| IBIS file stm32h562_563_573_lqfp64.ibs
[IBIS ver] 4.2
[File name] stm32h562_563_573_lqfp64.ibs
[File Rev] 1.1
[Date] 07-05-2024
[Source] Data Created at STMicroelectronics
[Notes]  File originated from ELDO simulations.
[Disclaimer]  This information is for modeling purpose only and is
   not guaranteed. The information is subject to change without
   notice.
[Copyright] Copyright 2024 STMicroelectronics Inc.
|   Component stm32h562_563_573_lqfp64
[Component] stm32h562_563_573_lqfp64
[Manufacturer] STMicroelectronics
[Package]
| variable   typ   min   max
R_pkg  0  NA  NA
L_pkg  0  NA  NA
C_pkg  0  NA  NA
[Pin]   signal_name   model_name
1  VBAT  power
2  PC13  io8_ft_i3c_spi
3  PC14-OSC32_IN  io8_ft_i3c_spi
4  PC15-OSC32_OUT  io8_ft_i3c_spi
5  PH0-OSC_IN  io8_ft_i3c_spi
6  PH1-OSC_OUT  io8_ft_i3c_spi
7  NRST  ioreset_ft_v33
8  PC0  io8_ft_spi
9  PC1  io8_ft_spi
10  PC2  io8_ft_spi
11  PC3  io8_ft_spi
12  VSSA  nc
13  VDDA  nc
14  PA0  io8_ft_spi
15  PA1  io8_ft_spi_tamp
16  PA2  io8_ft_spi
17  PA3  io8_ft_spi
18  VSS  gnd
19  VDD  power
20  PA4  io8_ft_spi
21  PA5  io8_ft_spi
22  PA6  io8_ft_spi
23  PA7  io8_ft_spi
24  PC4  io8_ft_spi
25  PC5  io8_ft_spi
26  PB0  io8_ft_spi
27  PB1  io8_ft_spi
28  PB2  io8_ft_i3c_spi
29  PB10  io8_ft_i3c_spi
30  VCAP  nc
31  VSS  gnd
32  VDD  power
33  PB12  io8_ft_i3c_spi
|34  PB13  io8usb_ft_pd
|35  PB14  io8usb_ft_pd
34 PB13 nc
35 PB14 nc
36  PB15  io8_ft_spi
37  PC6  io8_ft_i3c_spi
38  PC7  io8_ft_i3c_spi
39  PC8  io8_ft_i3c_spi
40  PC9  io8_ft_i3c_spi
41  PA8  io8_ft_i3c_spi
42  PA9  io8_ft_i3c_spi
43  PA10  io8_ft_i3c_spi
44  PA11  io8usb_ft_i3c_spi_phy
45  PA12  io8usb_ft_i3c_spi_phy
46  PA13  io8_ft_i3c_spi
47  VSS  gnd
48  VDD  power
49  PA14  io8_ft_i3c_spi
50  PA15  io8_ft_i3c_spi
51  PC10  io8_ft_i3c_spi
52  PC11  io8_ft_i3c_spi
53  PC12  io8_ft_i3c_spi
54  PD2  io8_ft_i3c_spi
55  PB3  io8_ft_i3c_spi
56  PB4  io8_ft_i3c_spi
57  PB5  io8_ft_i3c_spi
58  PB6  io8_ft_i3c_spi
59  PB7  io8_ft_i3c_spi
60  BOOT0  vpphv
61  PB8  io8_ft_i3c_spi
62  VCAP  nc
63  VSS  gnd
64  VDD  power
[Package Model]   484-lqfp-10x10-64-ldo-221014
[Pin Mapping]   pulldown_ref   pullup_ref   | Comment
1  nc  vsw
2  gndio  vddiom  | Depending on IO usage
| 2  gndio  vsw  | Depending on IO usage
3  gndio  vddiom  | Depending on IO usage
| 3  gndio  vsw  | Depending on IO usage
4  gndio  vddiom  | Depending on IO usage
| 4  gndio  vsw  | Depending on IO usage
5  gndio  vddiom
6  gndio  vddiom
7  gndio  vddiom
8  gndio  vddiom
9  gndio  vddiom
10  gndio  vddiom
11  gndio  vddiom
12  nc  nc
13  nc  nc
14  gndio  vddiom
15  gndio  vddiom
16  gndio  vddiom
17  gndio  vddiom
18  gndio  nc
19  nc  vddiom
20  gndio  vddiom
21  gndio  vddiom
22  gndio  vddiom
23  gndio  vddiom
24  gndio  vddiom
25  gndio  vddiom
26  gndio  vddiom
27  gndio  vddiom
28  gndio  vddiom
29  gndio  vddiom
30  nc  nc
31  gndio  nc
32  nc  vddiom
33  gndio  vddiom
|34  gndio  vddiom
|35  gndio  vddiom
34 nc nc
35 nc nc
36  gndio  vddiom
37  gndio  vddiom
38  gndio  vddiom
39  gndio  vddiom
40  gndio  vddiom
41  gndio  vddiom
42  gndio  vddiom
43  gndio  vddiom
44  gndio  vddiom
45  gndio  vddiom
46  gndio  vddiom
47  gndio  nc
48  nc  vddiom
49  gndio  vddiom
50  gndio  vddiom
51  gndio  vddiom
52  gndio  vddiom
53  gndio  vddiom
54  gndio  vddiom
55  gndio  vddiom
56  gndio  vddiom
57  gndio  vddiom
58  gndio  vddiom
59  gndio  vddiom
60  gndio  vddiom
61  gndio  vddiom
62  nc  nc
63  gndio  nc
64  nc  vddiom
[Model Selector] io8_ft_i3c_spi
io8_ft_spi_ls_1v2 "io8_ft spi low speed @ 1.2V"
io8_ft_spi_ls_1v8 "io8_ft spi low speed @ 1.8V"
io8_ft_spi_ls_3v3 "io8_ft spi low speed @ 3.3V"
io8_ft_spi_ms_1v2 "io8_ft spi med speed @ 1.2V"
io8_ft_spi_ms_1v8 "io8_ft spi med speed @ 1.8V"
io8_ft_spi_ms_3v3 "io8_ft spi med speed @ 3.3V"
io8_ft_spi_fs_1v2 "io8_ft spi fast speed @ 1.2V"
io8_ft_spi_fs_1v8 "io8_ft spi fast speed @ 1.8V"
io8_ft_spi_fs_3v3 "io8_ft spi fast speed @ 3.3V"
io8_ft_spi_hs_1v2 "io8_ft spi high speed @ 1.2V"
io8_ft_spi_hs_1v8 "io8_ft spi high speed @ 1.8V"
io8_ft_spi_hs_3v3 "io8_ft spi high speed @ 3.3V"
io8_ft_hslv_spi_ls_1v2 "io8_ft spi hslv low speed @ 1.2V"
io8_ft_hslv_spi_ls_1v8 "io8_ft spi hslv low speed @ 1.8V"
io8_ft_hslv_spi_ls_2v5 "io8_ft spi hslv low speed @ 2.5V"
io8_ft_hslv_spi_ms_1v2 "io8_ft spi hslv med speed @ 1.2V"
io8_ft_hslv_spi_ms_1v8 "io8_ft spi hslv med speed @ 1.8V"
io8_ft_hslv_spi_ms_2v5 "io8_ft spi hslv med speed @ 2.5V"
io8_ft_hslv_spi_fs_1v2 "io8_ft spi hslv fast speed @ 1.2V"
io8_ft_hslv_spi_fs_1v8 "io8_ft spi hslv fast speed @ 1.8V"
io8_ft_hslv_spi_fs_2v5 "io8_ft spi hslv fast speed @ 2.5V"
io8_ft_hslv_spi_hs_1v2 "io8_ft spi hslv high speed @ 1.2V"
io8_ft_hslv_spi_hs_1v8 "io8_ft spi hslv high speed @ 1.8V"
io8_ft_hslv_spi_hs_2v5 "io8_ft spi hslv high speed @ 2.5V"
io8_ft_i3c_spi_ls_1v2 "io8_ft i3c spi open-drain low speed @ 1.2V"
io8_ft_i3c_spi_ls_1v8 "io8_ft i3c spi open-drain low speed @ 1.8V"
io8_ft_i3c_spi_ls_3v3 "io8_ft i3c spi open-drain low speed @ 3.3V"
io8_ft_i3c_spi_ms_1v2 "io8_ft i3c spi open-drain med speed @ 1.2V"
io8_ft_i3c_spi_ms_1v8 "io8_ft i3c spi open-drain med speed @ 1.8V"
io8_ft_i3c_spi_ms_3v3 "io8_ft i3c spi open-drain med speed @ 3.3V"
io8_ft_i3c_spi_fs_1v2 "io8_ft i3c spi open-drain fast speed @ 1.2V"
io8_ft_i3c_spi_fs_1v8 "io8_ft i3c spi open-drain fast speed @ 1.8V"
io8_ft_i3c_spi_fs_3v3 "io8_ft i3c spi open-drain fast speed @ 3.3V"
io8_ft_i3c_spi_hs_1v2 "io8_ft i3c spi open-drain high speed @ 1.2V"
io8_ft_i3c_spi_hs_1v8 "io8_ft i3c spi open-drain high speed @ 1.8V"
io8_ft_i3c_spi_hs_3v3 "io8_ft i3c spi open-drain high speed @ 3.3V"
io8_ft_hslv_i3c_spi_ls_1v2 "io8_ft hslv i3c spi open-drain low speed @ 1.2V"
io8_ft_hslv_i3c_spi_ls_1v8 "io8_ft hslv i3c spi open-drain low speed @ 1.8V"
io8_ft_hslv_i3c_spi_ls_2v5 "io8_ft hslv i3c spi open-drain low speed @ 2.5V"
io8_ft_hslv_i3c_spi_ms_1v2 "io8_ft hslv i3c spi open-drain med speed @ 1.2V"
io8_ft_hslv_i3c_spi_ms_1v8 "io8_ft hslv i3c spi open-drain med speed @ 1.8V"
io8_ft_hslv_i3c_spi_ms_2v5 "io8_ft hslv i3c spi open-drain med speed @ 2.5V"
io8_ft_hslv_i3c_spi_fs_1v2 "io8_ft hslv i3c spi open-drain fast speed @ 1.2V"
io8_ft_hslv_i3c_spi_fs_1v8 "io8_ft hslv i3c spi open-drain fast speed @ 1.8V"
io8_ft_hslv_i3c_spi_fs_2v5 "io8_ft hslv i3c spi open-drain fast speed @ 2.5V"
io8_ft_hslv_i3c_spi_hs_1v2 "io8_ft hslv i3c spi open-drain high speed @ 1.2V"
io8_ft_hslv_i3c_spi_hs_1v8 "io8_ft hslv i3c spi open-drain high speed @ 1.8V"
io8_ft_hslv_i3c_spi_hs_2v5 "io8_ft hslv i3c spi open-drain high speed @ 2.5V"
io8_ft_i3c_fmp_spi_3v3 "io8_ft i3c fm+ spi open-drain @ 3.3V"
io8_ft_i3c_fmp_spi_1v8 "io8_ft i3c fm+ spi open-drain @ 1.8V"
io8_ft_i3c_fmp_spi_1v2 "io8_ft i3c fm+ spi open-drain @ 1.2V"
[Model Selector] io8_ft_spi
io8_ft_spi_ls_1v2 "io8_ft spi low speed @ 1.2V"
io8_ft_spi_ls_1v8 "io8_ft spi low speed @ 1.8V"
io8_ft_spi_ls_3v3 "io8_ft spi low speed @ 3.3V"
io8_ft_spi_ms_1v2 "io8_ft spi med speed @ 1.2V"
io8_ft_spi_ms_1v8 "io8_ft spi med speed @ 1.8V"
io8_ft_spi_ms_3v3 "io8_ft spi med speed @ 3.3V"
io8_ft_spi_fs_1v2 "io8_ft spi fast speed @ 1.2V"
io8_ft_spi_fs_1v8 "io8_ft spi fast speed @ 1.8V"
io8_ft_spi_fs_3v3 "io8_ft spi fast speed @ 3.3V"
io8_ft_spi_hs_1v2 "io8_ft spi high speed @ 1.2V"
io8_ft_spi_hs_1v8 "io8_ft spi high speed @ 1.8V"
io8_ft_spi_hs_3v3 "io8_ft spi high speed @ 3.3V"
io8_ft_hslv_spi_ls_1v2 "io8_ft spi hslv low speed @ 1.2V"
io8_ft_hslv_spi_ls_1v8 "io8_ft spi hslv low speed @ 1.8V"
io8_ft_hslv_spi_ls_2v5 "io8_ft spi hslv low speed @ 2.5V"
io8_ft_hslv_spi_ms_1v2 "io8_ft spi hslv med speed @ 1.2V"
io8_ft_hslv_spi_ms_1v8 "io8_ft spi hslv med speed @ 1.8V"
io8_ft_hslv_spi_ms_2v5 "io8_ft spi hslv med speed @ 2.5V"
io8_ft_hslv_spi_fs_1v2 "io8_ft spi hslv fast speed @ 1.2V"
io8_ft_hslv_spi_fs_1v8 "io8_ft spi hslv fast speed @ 1.8V"
io8_ft_hslv_spi_fs_2v5 "io8_ft spi hslv fast speed @ 2.5V"
io8_ft_hslv_spi_hs_1v2 "io8_ft spi hslv high speed @ 1.2V"
io8_ft_hslv_spi_hs_1v8 "io8_ft spi hslv high speed @ 1.8V"
io8_ft_hslv_spi_hs_2v5 "io8_ft spi hslv high speed @ 2.5V"
[Model Selector] io8_ft_spi_tamp
io8_ft_spi_ls_1v2 "io8_ft spi low speed @ 1.2V"
io8_ft_spi_ls_1v8 "io8_ft spi low speed @ 1.8V"
io8_ft_spi_ls_3v3 "io8_ft spi low speed @ 3.3V"
io8_ft_spi_ms_1v2 "io8_ft spi med speed @ 1.2V"
io8_ft_spi_ms_1v8 "io8_ft spi med speed @ 1.8V"
io8_ft_spi_ms_3v3 "io8_ft spi med speed @ 3.3V"
io8_ft_spi_fs_1v2 "io8_ft spi fast speed @ 1.2V"
io8_ft_spi_fs_1v8 "io8_ft spi fast speed @ 1.8V"
io8_ft_spi_fs_3v3 "io8_ft spi fast speed @ 3.3V"
io8_ft_spi_hs_1v2 "io8_ft spi high speed @ 1.2V"
io8_ft_spi_hs_1v8 "io8_ft spi high speed @ 1.8V"
io8_ft_spi_hs_3v3 "io8_ft spi high speed @ 3.3V"
io8_ft_hslv_spi_ls_1v2 "io8_ft spi hslv low speed @ 1.2V"
io8_ft_hslv_spi_ls_1v8 "io8_ft spi hslv low speed @ 1.8V"
io8_ft_hslv_spi_ls_2v5 "io8_ft spi hslv low speed @ 2.5V"
io8_ft_hslv_spi_ms_1v2 "io8_ft spi hslv med speed @ 1.2V"
io8_ft_hslv_spi_ms_1v8 "io8_ft spi hslv med speed @ 1.8V"
io8_ft_hslv_spi_ms_2v5 "io8_ft spi hslv med speed @ 2.5V"
io8_ft_hslv_spi_fs_1v2 "io8_ft spi hslv fast speed @ 1.2V"
io8_ft_hslv_spi_fs_1v8 "io8_ft spi hslv fast speed @ 1.8V"
io8_ft_hslv_spi_fs_2v5 "io8_ft spi hslv fast speed @ 2.5V"
io8_ft_hslv_spi_hs_1v2 "io8_ft spi hslv high speed @ 1.2V"
io8_ft_hslv_spi_hs_1v8 "io8_ft spi hslv high speed @ 1.8V"
io8_ft_hslv_spi_hs_2v5 "io8_ft spi hslv high speed @ 2.5V"
io8_ft_tamp_v33_1v2 "io8_ft tamp V33 @ 1.2V"
io8_ft_tamp_v33_1v8 "io8_ft tamp V33 @ 1.2V"
io8_ft_tamp_v33_3v3 "io8_ft tamp V33 @ 1.2V"
[Model Selector] io8usb_ft_i3c_spi_phy
io8_ft_spi_ls_1v2 "io8_ft spi low speed @ 1.2V"
io8_ft_spi_ls_1v8 "io8_ft spi low speed @ 1.8V"
io8_ft_spi_ls_3v3 "io8_ft spi low speed @ 3.3V"
io8_ft_spi_ms_1v2 "io8_ft spi med speed @ 1.2V"
io8_ft_spi_ms_1v8 "io8_ft spi med speed @ 1.8V"
io8_ft_spi_ms_3v3 "io8_ft spi med speed @ 3.3V"
io8_ft_spi_fs_1v2 "io8_ft spi fast speed @ 1.2V"
io8_ft_spi_fs_1v8 "io8_ft spi fast speed @ 1.8V"
io8_ft_spi_fs_3v3 "io8_ft spi fast speed @ 3.3V"
io8_ft_spi_hs_1v2 "io8_ft spi high speed @ 1.2V"
io8_ft_spi_hs_1v8 "io8_ft spi high speed @ 1.8V"
io8_ft_spi_hs_3v3 "io8_ft spi high speed @ 3.3V"
io8_ft_hslv_spi_ls_1v2 "io8_ft spi hslv low speed @ 1.2V"
io8_ft_hslv_spi_ls_1v8 "io8_ft spi hslv low speed @ 1.8V"
io8_ft_hslv_spi_ls_2v5 "io8_ft spi hslv low speed @ 2.5V"
io8_ft_hslv_spi_ms_1v2 "io8_ft spi hslv med speed @ 1.2V"
io8_ft_hslv_spi_ms_1v8 "io8_ft spi hslv med speed @ 1.8V"
io8_ft_hslv_spi_ms_2v5 "io8_ft spi hslv med speed @ 2.5V"
io8_ft_hslv_spi_fs_1v2 "io8_ft spi hslv fast speed @ 1.2V"
io8_ft_hslv_spi_fs_1v8 "io8_ft spi hslv fast speed @ 1.8V"
io8_ft_hslv_spi_fs_2v5 "io8_ft spi hslv fast speed @ 2.5V"
io8_ft_hslv_spi_hs_1v2 "io8_ft spi hslv high speed @ 1.2V"
io8_ft_hslv_spi_hs_1v8 "io8_ft spi hslv high speed @ 1.8V"
io8_ft_hslv_spi_hs_2v5 "io8_ft spi hslv high speed @ 2.5V"
io8_ft_i3c_spi_ls_1v2 "io8_ft i3c spi open-drain low speed @ 1.2V"
io8_ft_i3c_spi_ls_1v8 "io8_ft i3c spi open-drain low speed @ 1.8V"
io8_ft_i3c_spi_ls_3v3 "io8_ft i3c spi open-drain low speed @ 3.3V"
io8_ft_i3c_spi_ms_1v2 "io8_ft i3c spi open-drain med speed @ 1.2V"
io8_ft_i3c_spi_ms_1v8 "io8_ft i3c spi open-drain med speed @ 1.8V"
io8_ft_i3c_spi_ms_3v3 "io8_ft i3c spi open-drain med speed @ 3.3V"
io8_ft_i3c_spi_fs_1v2 "io8_ft i3c spi open-drain fast speed @ 1.2V"
io8_ft_i3c_spi_fs_1v8 "io8_ft i3c spi open-drain fast speed @ 1.8V"
io8_ft_i3c_spi_fs_3v3 "io8_ft i3c spi open-drain fast speed @ 3.3V"
io8_ft_i3c_spi_hs_1v2 "io8_ft i3c spi open-drain high speed @ 1.2V"
io8_ft_i3c_spi_hs_1v8 "io8_ft i3c spi open-drain high speed @ 1.8V"
io8_ft_i3c_spi_hs_3v3 "io8_ft i3c spi open-drain high speed @ 3.3V"
io8_ft_hslv_i3c_spi_ls_1v2 "io8_ft hslv i3c spi open-drain low speed @ 1.2V"
io8_ft_hslv_i3c_spi_ls_1v8 "io8_ft hslv i3c spi open-drain low speed @ 1.8V"
io8_ft_hslv_i3c_spi_ls_2v5 "io8_ft hslv i3c spi open-drain low speed @ 2.5V"
io8_ft_hslv_i3c_spi_ms_1v2 "io8_ft hslv i3c spi open-drain med speed @ 1.2V"
io8_ft_hslv_i3c_spi_ms_1v8 "io8_ft hslv i3c spi open-drain med speed @ 1.8V"
io8_ft_hslv_i3c_spi_ms_2v5 "io8_ft hslv i3c spi open-drain med speed @ 2.5V"
io8_ft_hslv_i3c_spi_fs_1v2 "io8_ft hslv i3c spi open-drain fast speed @ 1.2V"
io8_ft_hslv_i3c_spi_fs_1v8 "io8_ft hslv i3c spi open-drain fast speed @ 1.8V"
io8_ft_hslv_i3c_spi_fs_2v5 "io8_ft hslv i3c spi open-drain fast speed @ 2.5V"
io8_ft_hslv_i3c_spi_hs_1v2 "io8_ft hslv i3c spi open-drain high speed @ 1.2V"
io8_ft_hslv_i3c_spi_hs_1v8 "io8_ft hslv i3c spi open-drain high speed @ 1.8V"
io8_ft_hslv_i3c_spi_hs_2v5 "io8_ft hslv i3c spi open-drain high speed @ 2.5V"
io8_ft_i3c_fmp_spi_3v3 "io8_ft i3c fm+ spi open-drain @ 3.3V"
io8_ft_i3c_fmp_spi_1v8 "io8_ft i3c fm+ spi open-drain @ 1.8V"
io8_ft_i3c_fmp_spi_1v2 "io8_ft i3c fm+ spi open-drain @ 1.2V"
io8usb_ft_phy_ls_2v5 "iousb ft low speed @ 2.5V"
io8usb_ft_phy_ls_3v3 "iousb ft low speed @ 3.3V"
io8usb_ft_phy_fs_2v5 "iousb ft fast speed @ 2.5V"
io8usb_ft_phy_fs_3v3 "iousb ft fast speed @ 3.3V"
[Model Selector] ioreset_ft_v33
ioreset_ft_v33_1v2 "Reset PAD. 5V tolerant. 1.2V range"
ioreset_ft_v33_1v8 "Reset PAD. 5V tolerant. 1.8V range"
ioreset_ft_v33_3v3 "Reset PAD. 5V tolerant. 3.3V range"
[Model Selector] vpphv
vpphv_1v2 "Flash Test cell v33 = 1.2 V range"
vpphv_1v8 "Flash Test cell v33 = 1.8 V range"
vpphv_3v3 "Flash Test cell v33 = 3.3 V range"
[Define Package Model]  484-lqfp-10x10-64-ldo-221014
[Manufacturer]  Unknown
[OEM]  Unknown
[Description]  None
[Number Of Pins]  61
[Pin Numbers]
| Pin Num   Terminal Name
7 | NRST
14 | PA0
15 | PA1
16 | PA2
17 | PA3
20 | PA4
21 | PA5
22 | PA6
23 | PA7
41 | PA8
42 | PA9
43 | PA10
44 | PA11
45 | PA12
46 | PA13
49 | PA14
50 | PA15
26 | PB0
27 | PB1
28 | PB2
55 | PB3
56 | PB4
57 | PB5
58 | PB6
59 | PB7
61 | PB8
29 | PB10
33 | PB12
34 | PB13
35 | PB14
36 | PB15
8 | PC0
9 | PC1
10 | PC2
11 | PC3
24 | PC4
25 | PC5
37 | PC6
38 | PC7
39 | PC8
40 | PC9
51 | PC10
52 | PC11
53 | PC12
2 | PC13
3 | PC14-OSC32_IN
4 | PC15-OSC32_OUT
54 | PD2
5 | PH0-OSC_IN
6 | PH1-OSC_OUT
1 | VBAT
30 | VCAP
62 | VCAP
32 | VDD
48 | VDD
19 | VDD
64 | VDD
13 | VDDA
60 | BOOT0
18 | VSS
12 | VSSA
|[Merged Pins]  18
|31  |  VSS
|47  |  VSS
|63  |  VSS
[Model Data]
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[End Model Data]
[End Package Model]
|End [Component]
| Models and submodels in the file (64): io8_ft_hslv_i3c_spi_fs_1v2 (I/O_open_drain), io8_ft_hslv_i3c_spi_fs_1v8 (I/O_open_drain), io8_ft_hslv_i3c_spi_fs_2v5 (I/O_open_drain), io8_ft_hslv_i3c_spi_hs_1v2 (I/O_open_drain), io8_ft_hslv_i3c_spi_hs_1v8 (I/O_open_drain), io8_ft_hslv_i3c_spi_hs_2v5 (I/O_open_drain), io8_ft_hslv_i3c_spi_ls_1v2 (I/O_open_drain), io8_ft_hslv_i3c_spi_ls_1v8 (I/O_open_drain), io8_ft_hslv_i3c_spi_ls_2v5 (I/O_open_drain), io8_ft_hslv_i3c_spi_ms_1v2 (I/O_open_drain), io8_ft_hslv_i3c_spi_ms_1v8 (I/O_open_drain), io8_ft_hslv_i3c_spi_ms_2v5 (I/O_open_drain), io8_ft_hslv_spi_fs_1v2 (I/O), io8_ft_hslv_spi_fs_1v8 (I/O), io8_ft_hslv_spi_fs_2v5 (I/O), io8_ft_hslv_spi_hs_1v2 (I/O), io8_ft_hslv_spi_hs_1v8 (I/O), io8_ft_hslv_spi_hs_2v5 (I/O), io8_ft_hslv_spi_ls_1v2 (I/O), io8_ft_hslv_spi_ls_1v8 (I/O), io8_ft_hslv_spi_ls_2v5 (I/O), io8_ft_hslv_spi_ms_1v2 (I/O), io8_ft_hslv_spi_ms_1v8 (I/O), io8_ft_hslv_spi_ms_2v5 (I/O), io8_ft_i3c_fmp_spi_1v2 (I/O_open_drain), io8_ft_i3c_fmp_spi_1v8 (I/O_open_drain), io8_ft_i3c_fmp_spi_3v3 (I/O_open_drain), io8_ft_i3c_spi_fs_1v2 (I/O_open_drain), io8_ft_i3c_spi_fs_1v8 (I/O_open_drain), io8_ft_i3c_spi_fs_3v3 (I/O_open_drain), io8_ft_i3c_spi_hs_1v2 (I/O_open_drain), io8_ft_i3c_spi_hs_1v8 (I/O_open_drain), io8_ft_i3c_spi_hs_3v3 (I/O_open_drain), io8_ft_i3c_spi_ls_1v2 (I/O_open_drain), io8_ft_i3c_spi_ls_1v8 (I/O_open_drain), io8_ft_i3c_spi_ls_3v3 (I/O_open_drain), io8_ft_i3c_spi_ms_1v2 (I/O_open_drain), io8_ft_i3c_spi_ms_1v8 (I/O_open_drain), io8_ft_i3c_spi_ms_3v3 (I/O_open_drain), io8_ft_spi_fs_1v2 (I/O), io8_ft_spi_fs_1v8 (I/O), io8_ft_spi_fs_3v3 (I/O), io8_ft_spi_hs_1v2 (I/O), io8_ft_spi_hs_1v8 (I/O), io8_ft_spi_hs_3v3 (I/O), io8_ft_spi_ls_1v2 (I/O), io8_ft_spi_ls_1v8 (I/O), io8_ft_spi_ls_3v3 (I/O), io8_ft_spi_ms_1v2 (I/O), io8_ft_spi_ms_1v8 (I/O), io8_ft_spi_ms_3v3 (I/O), io8_ft_tamp_v33_1v2 (I/O), io8_ft_tamp_v33_1v8 (I/O), io8_ft_tamp_v33_3v3 (I/O), io8usb_ft_phy_fs_2v5 (I/O), io8usb_ft_phy_fs_3v3 (I/O), io8usb_ft_phy_ls_2v5 (I/O), io8usb_ft_phy_ls_3v3 (I/O), ioreset_ft_v33_1v2 (I/O_open_drain), ioreset_ft_v33_1v8 (I/O_open_drain), ioreset_ft_v33_3v3 (I/O_open_drain), vpphv_1v2 (Input), vpphv_1v8 (Input), vpphv_3v3 (Input)
